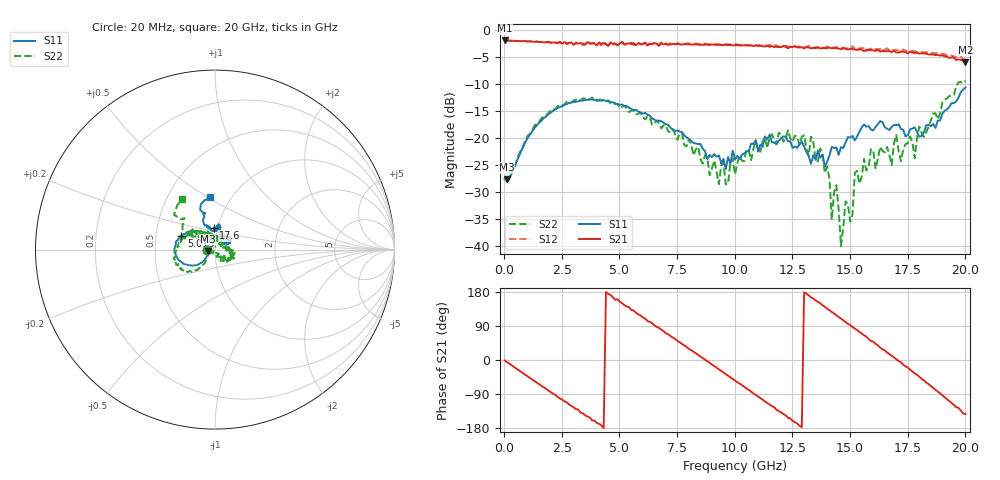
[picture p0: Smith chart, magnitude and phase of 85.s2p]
!Agilent Technologies,N5230A,US43500223,A.07.50.48
!Agilent N5230A: A.07.50.48
!Date: Sunday, September 13, 2015 20:59:13
!Correction: S11(Full 2 Port(1,2))
!S21(Full 2 Port(1,2))
!S12(Full 2 Port(1,2))
!S22(Full 2 Port(1,2))
!S2P File: Measurements: S11, S21, S12, S22:
# Hz S  dB  R 50
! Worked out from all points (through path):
!   201 points, 20 MHz to 20 GHz, reference 50 ohm
!   highest |S21| = -2.01 dB at 20 MHz (marker M1); lowest = -6.0 dB at 20 GHz (marker M2)
!   group delay of S21, straight-line fit = 118 ps
!   lowest |S11| = -27.7 dB at 119.9 MHz (marker M3), VSWR 1.09, Z = 46.1 - j0.664 ohm
!   |S11| at or under -10 dB: start of sweep to end of sweep
!   |S22| runs from -40.0 to -9.4 dB; largest |S21 - S12| = 0.05
!   S11 on the Smith chart (normalised r, x): 20 MHz: 0.92, +0.00; 5.015 GHz: 0.68, +0.11; 17.6 GHz: 0.96, +0.23; 20 GHz: 0.80, +0.51
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2e7  -27.49 179.8  -2.01 -1.0  -2.01 -1.0  -27.47 -179.2
1.199e8  -27.67 -170.0  -2.03 -5.2  -2.02 -5.3  -28.05 -167.7
1.9181e9  -15.60 -147.8  -2.25 -80.6  -2.25 -81.0  -15.42 -134.7
3.4166e9  -13.10 -175.3  -2.59 -140.8  -2.88 -140.4  -12.67 -158.9
5.015e9  -13.88 157.6  -2.59 153.7  -2.42 153.2  -14.50 168.2
6.7133e9  -16.79 133.0  -3.01 84.6  -2.83 83.8  -17.31 130.1
8.4116e9  -21.13 117.9  -2.80 13.3  -2.63 12.5  -21.65 91.8
1.001e10  -23.98 86.8  -2.87 -54.0  -2.75 -54.6  -26.73 13.5
1.15085e10  -19.41 38.5  -3.19 -117.5  -2.78 -119.1  -19.96 -2.0
1.34066e10  -23.16 39.8  -3.38 162.1  -3.35 161.0  -20.79 -50.8
1.4006e10  -24.39 56.1  -3.41 135.5  -3.10 135.7  -25.27 -44.3
1.42058e10  -21.65 62.4  -3.45 126.6  -3.32 127.1  -35.11 -93.1
1.44056e10  -21.74 58.2  -3.42 118.2  -3.22 116.8  -28.71 -64.6
1.46054e10  -21.71 70.0  -3.62 109.5  -3.40 108.7  -39.98 153.7
1.48052e10  -20.82 71.8  -3.54 99.8  -3.51 98.4  -31.70 -145.8
1.51049e10  -19.61 70.6  -3.62 86.8  -3.07 85.9  -34.19 -175.1
1.52048e10  -20.47 69.6  -3.69 82.9  -3.51 80.8  -26.47 160.6
1.67033e10  -18.54 83.7  -3.95 15.7  -3.86 13.8  -23.16 107.0
1.76024e10  -18.40 93.8  -4.09 -25.6  -3.96 -26.5  -19.72 125.5
1.78022e10  -18.03 90.5  -4.34 -35.4  -4.00 -36.9  -23.74 130.8
1.88012e10  -16.79 108.8  -4.71 -83.4  -4.34 -85.8  -16.55 140.4
2e10  -10.69 95.9  -6.00 -142.4  -5.76 -145.9  -9.45 123.4
